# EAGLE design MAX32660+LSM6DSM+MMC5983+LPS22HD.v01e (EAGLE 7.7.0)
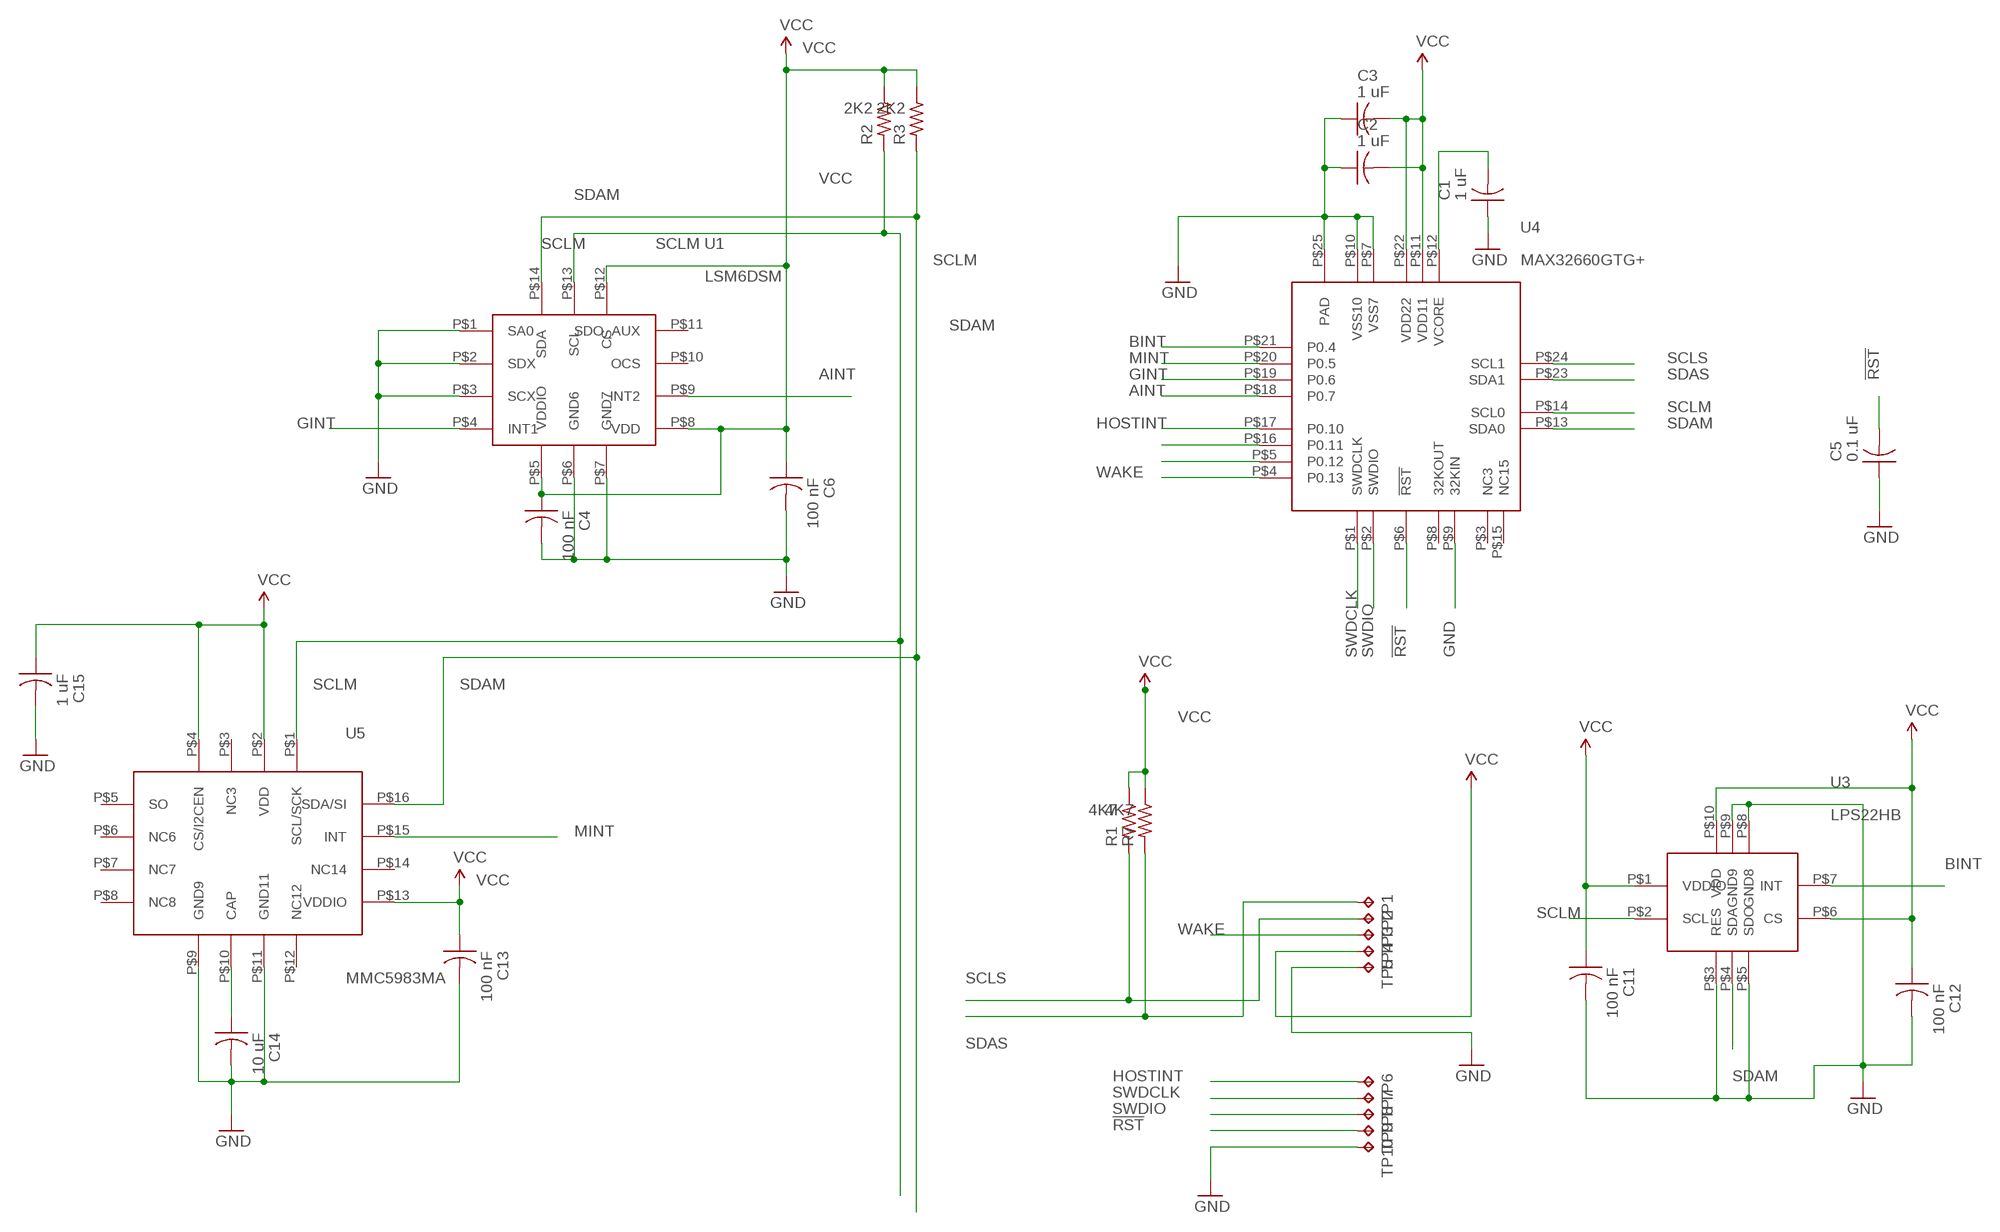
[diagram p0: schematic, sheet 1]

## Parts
C1  1 uF  C-US  [C0402_B]
C2  1 uF  C-US  [C0402_B]
C3  1 uF  C-US  [C0402_B]
C4  100 nF  C-US  [C0402_B]
C5  0.1 uF  C-US  [C0402_B]
C6  100 nF  C-US  [C0402_B]
C11  100 nF  C-US  [C0402_B]
C12  100 nF  C-US  [C0402_B]
C13  100 nF  C-US  [C0402_B]
C14  10 uF  C-US  [C0402_B]
C15  1 uF  C-US  [C0402_B]
R1  4K7  R-US_  [R0402_B]
R2  2K2  R-US_  [R0402_B]
R3  2K2  R-US_  [R0402_B]
R7  4K7  R-US_  [R0402_B]
TP1  TPTP08SQ  [TP08SQ]
TP2  TPTP08SQ  [TP08SQ]
TP3  TPTP08SQ  [TP08SQ]
TP4  TPTP08SQ  [TP08SQ]
TP5  TPTP08SQ  [TP08SQ]
TP6  TPTP08SQ  [TP08SQ]
TP7  TPTP08SQ  [TP08SQ]
TP8  TPTP08SQ  [TP08SQ]
TP9  TPTP08SQ  [TP08SQ]
TP10  TPTP08SQ  [TP08SQ]
U1  LSM6DSM  [LSM6DSM]
U3  LPS22HB  [LPS22HB]
U4  MAX32660GTG+  [MAX32660GTG+]
U5  MMC5983MA  [MMC5983MA]

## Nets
!RST: C5.2 TP9.TP U4.P$6(!RST)
AINT: U1.P$9(INT2) U4.P$18(P0.7)
BINT: U3.P$7(INT) U4.P$21(P0.4)
GINT: U1.P$4(INT1) U4.P$19(P0.6)
GND: C1.1 C2.1 C3.1 C4.2 C5.1 C6.2 C11.2 C12.2 C13.2 C14.2 C15.2 TP5.TP TP10.TP U1.P$1(SA0) U1.P$2(SDX) U1.P$3(SCX) U1.P$6(GND6) U1.P$7(GND7) U3.P$3(RES) U3.P$5(SDO) U3.P$8(GND8) U3.P$9(GND9) U4.P$7(VSS7) U4.P$9(32KIN) U4.P$10(VSS10) U4.P$25(PAD) U5.P$9(GND9) U5.P$11(GND11)
HOSTINT: TP6.TP U4.P$17(P0.10)
MINT: U4.P$20(P0.5) U5.P$15(INT)
N$2: C14.1 U5.P$10(CAP)
N$6: C1.2 U4.P$12(VCORE)
N$8: U4.P$16(P0.11)
N$9: U4.P$5(P0.12)
SCLM: R2.2 U1.P$13(SCL) U3.P$2(SCL) U4.P$14(SCL0) U5.P$1(SCL/SCK)
SCLS: R1.2 TP2.TP U4.P$24(SCL1)
SDAM: R3.2 U1.P$14(SDA) U3.P$4(SDA) U4.P$13(SDA0) U5.P$16(SDA/SI)
SDAS: R7.2 TP1.TP U4.P$23(SDA1)
SWDCLK: TP7.TP U4.P$1(SWDCLK)
SWDIO: TP8.TP U4.P$2(SWDIO)
VCC: C2.2 C3.2 C4.1 C6.1 C11.1 C12.1 C13.1 C15.1 R1.1 R2.1 R3.1 R7.1 TP4.TP U1.P$5(VDDIO) U1.P$8(VDD) U1.P$12(CS) U3.P$1(VDDIO) U3.P$6(CS) U3.P$10(VDD) U4.P$11(VDD11) U4.P$22(VDD22) U5.P$2(VDD) U5.P$4(CS/I2CEN) U5.P$13(VDDIO)
WAKE: TP3.TP U4.P$4(P0.13)
Unconnected: U4.P$3(NC3) U4.P$8(32KOUT) U4.P$15(NC15) U5.P$3(NC3) U5.P$5(SO) U5.P$6(NC6) U5.P$7(NC7) U5.P$8(NC8) U5.P$12(NC12) U5.P$14(NC14)

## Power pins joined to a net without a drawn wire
OCS: U1.P$10(OCS)
SDO_AUX: U1.P$11(SDO_AUX)

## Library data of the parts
C1-C6 C11-C15 = Spark:C-US: Capacitor
R1-R3 R7 = Spark:R-US_: 0402 Resistor
TP1-TP10 = testpad:TP: Test pad
U1 = Kris:LSM6DSM: LSM6DSM ST accel/gyro
U3 = Kris:LPS22HB: LPS22HB ST pressure sensor http://www.st.com/content/ccc/resource/technical/document/datasheet/bf/c1/4f/23/61/17/44/8a/DM00140895.pdf/files/DM00140895.pdf/jcr:content/translations/en.DM00140895.pdf
U4 = Kris:MAX32660GTG+: MAX32660GTG+ 3 mm x 3 mm 24-pin TQFN package https://pdfserv.maximintegrated.com/land_patterns/90-100089.PDF https://datasheets.maximintegrated.com/en/ds/MAX32660.pdf
U5 = Kris:MMC5983MA: MMC5983MA ±8 Gauss, High Performance 3-axis Magnetic Sensor https://www.mouser.com/datasheet/2/821/Memsic_09102019_MMC5983MA_Datasheet_Rev_A-1635338.pdf

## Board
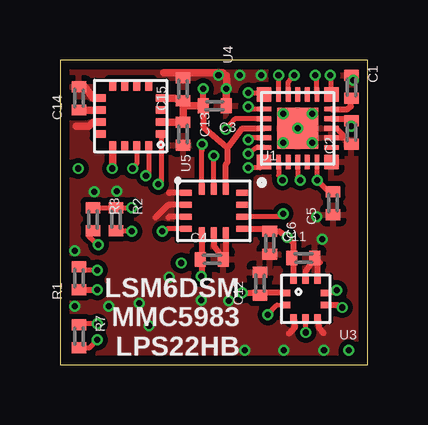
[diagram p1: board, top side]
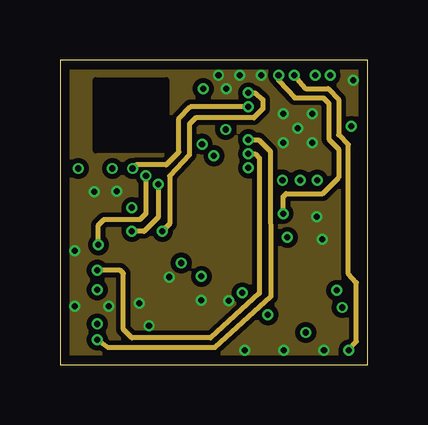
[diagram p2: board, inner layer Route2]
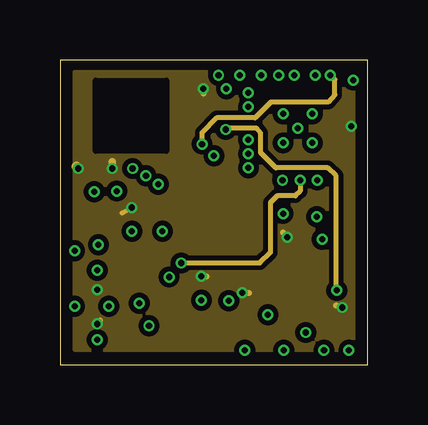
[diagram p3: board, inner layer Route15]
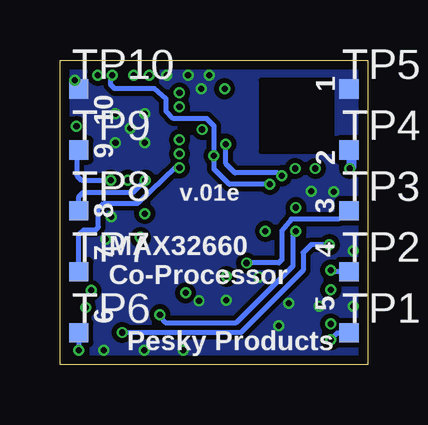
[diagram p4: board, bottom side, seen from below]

Size 12.83 x 12.7 mm. Coordinates in mm from the lower left corner, seen from the top.
Outline: 0,0 12.83,0 12.83,12.7 0,12.7 0,0
Copper layers (1*2*15*16): Top 0.035559375mm / dielectric 0.17018125mm / Route2 0.01778125mm / dielectric 47mil / Route15 0.01778125mm / dielectric 0.17018125mm / Bottom 0.035559375mm
Design rules "OSHPark-4layer *": minimum track width 5mil, minimum drill 10mil, track to track 5mil, track to pad 5mil, pad to pad 5mil, via to via 5mil, smd to smd 5mil, copper to edge 15mil, drill to drill 6mil, minimum pad ring 4mil, minimum via ring 4mil, stop-mask expansion 4mil, vias tented up to drill 20mil, thermal gap 10mil

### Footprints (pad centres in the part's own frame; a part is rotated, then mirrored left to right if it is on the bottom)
C0402_B = smd 0.457 x 0.61: 1 -0.483,0; 2 0.483,0
R0402_B = smd 0.457 x 0.61: 1 -0.483,0; 2 0.483,0
TP08SQ = smd 0.8 x 0.8: TP 0,0
LSM6DSM = smd 0.475 x 0.25: P$1 -1.163,0.75; P$2 -1.163,0.25; P$3 -1.163,-0.25; P$4 -1.163,-0.75; P$8 1.163,-0.75; P$9 1.163,-0.25; P$10 1.163,0.25; P$11 1.163,0.75 | smd 0.25 x 0.475: P$5 -0.5,-0.912; P$6 0,-0.912; P$7 0.5,-0.912; P$12 0.5,0.912; P$13 0,0.912; P$14 -0.5,0.912
LPS22HB = smd 0.3 x 0.275: P$1 -0.787,0.25; P$2 -0.787,-0.25; P$6 0.787,-0.25; P$7 0.787,0.25 | smd 0.275 x 0.3: P$3 -0.5,-0.787; P$4 0,-0.787; P$5 0.5,-0.787; P$8 0.5,0.787; P$9 0,0.787; P$10 -0.5,0.787
MAX32660GTG+ = smd 0.6 x 0.6: P$1 -1.4,1.4; P$7 -1.4,-1.4; P$13 1.4,-1.4; P$19 1.4,1.4 | smd 0.6 x 0.2: P$2 -1.4,0.8; P$3 -1.4,0.4; P$4 -1.4,0; P$5 -1.4,-0.4; P$6 -1.4,-0.8; P$14 1.4,-0.8; P$15 1.4,-0.4; P$16 1.4,0; P$17 1.4,0.4; P$18 1.4,0.8 | smd 0.2 x 0.6: P$8 -0.8,-1.4; P$9 -0.4,-1.4; P$10 0,-1.4; P$11 0.4,-1.4; P$12 0.8,-1.4; P$20 0.8,1.4; P$21 0.4,1.4; P$22 0,1.4; P$23 -0.4,1.4; P$24 -0.8,1.4 | smd 1.7 x 1.7: P$25 0,0
MMC5983MA = smd 0.3 x 0.45: P$1 0.75,1.275; P$2 0.25,1.275; P$3 -0.25,1.275; P$4 -0.75,1.275; P$9 -0.75,-1.275; P$10 -0.25,-1.275; P$11 0.25,-1.275; P$12 0.75,-1.275 | smd 0.45 x 0.3: P$5 -1.275,0.75; P$6 -1.275,0.25; P$7 -1.275,-0.25; P$8 -1.275,-0.75; P$13 1.275,-0.75; P$14 1.275,-0.25; P$15 1.275,0.25; P$16 1.275,0.75

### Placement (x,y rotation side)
C1  12.14,11.58 270 top
C2  12.14,9.68 90 top
C3  6.45,10.79 180 top
C4  6.32,4.39 0 top
C5  11.38,6.73 90 top
C6  8.74,5.08 270 top
C11  10.13,4.45 0 top
C12  8.33,3.38 90 top
C13  5.13,9.63 270 top
C14  0.79,11.1 90 top
C15  5.13,11.48 90 top
R1  0.79,3.61 90 top
R2  2.34,6.07 270 top
R3  1.37,6.07 270 top
R7  0.79,1.19 270 top
TP1  0.79,1.33 0 bottom
TP2  0.79,3.87 0 bottom
TP3  0.79,6.41 0 bottom
TP4  0.79,8.95 0 bottom
TP5  0.79,11.49 0 bottom
TP6  12.04,1.33 0 bottom
TP7  12.04,3.87 0 bottom
TP8  12.04,6.41 0 bottom
TP9  12.04,8.95 0 bottom
TP10  12.04,11.49 0 bottom
U1  6.41,6.41 0 top
U3  10.24,2.74 0 top
U4  9.91,9.86 90 top
U5  2.95,10.36 270 top

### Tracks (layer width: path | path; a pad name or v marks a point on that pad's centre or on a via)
!RST  (via drill 0.25)
  Top 0.203: U4.P$6 10.71,7.89 v10.72,7.7 11.2,7.21 C5.2
  Bottom 0.203: TP9.TP 12.13,8.97 12.13,7.89 11.94,7.7 v10.72,7.7
AINT  (via drill 0.25)
  Top 0.203: U4.P$18 v9.11,12.06 | v9.3,6.3 9.17,6.17 7.58,6.17 U1.P$9
  Route2 0.203: 9.4,6.3 v9.3,6.3 9.3,7.01 9.42,7.14 10.95,7.14 11.61,7.8 11.61,8.99 11.2,9.4 11.2,10.9 10.97,11.12 9.78,11.12 9.11,11.84 v9.11,12.06
BINT  (via drill 0.25)
  Top 0.203: U4.P$21 7.31,10.26 v6.91,9.8 | v11.53,3.1 11.53,3 11.18,3 11.18,2.99 U3.P$7
  Route15 0.203: v11.53,3.1 11.51,3.28 11.51,7.87 11.15,8.2 8.99,8.2 8.36,8.84 8.36,9.65 8.2,9.86 6.96,9.86 v6.91,9.8
GINT  (via drill 0.25)
  Top 0.203: U1.P$4 4.47,5.66 v4.27,5.56 | v7.85,11.33 8.38,11.33 U4.P$19
  Route2 0.203: v7.85,11.33 8.13,11.33 8.45,11.05 8.45,10.66 8.08,10.29 5.65,10.29 5.39,10.03 5.39,8.74 4.57,7.87 4.57,5.87 v4.27,5.56
GND  (via drill 0.25)
  Top 0.203: U4.P$9 11.91,9.46 | 10.85,4.27 C11.2 | U4.P$10 11.51,9.86 11.91,9.46 | 11.91,9.46 11.98,9.38 C2.1
  Top 0.254: U1.P$3 4.54,6.16 4.52,6.15 | 4.55,6.68 4.56,6.66 U1.P$2 4.5,6.66 3.99,6.15 | U1.P$1 4.57,7.16 4.55,7.19 | U1.P$6 6.41,4.97 C4.2 6.91,4.6 U1.P$7 | U3.P$9 10.24,3.89 C11.2 10.74,4.25 U3.P$8 | U3.P$5 10.79,1.56 10.97,1.32 | U3.P$3 9.79,1.56 9.55,1.29
  Top 0.305: U5.P$11 1.38,10.11 1.19,9.93 0.69,9.93 | C3.1 v6.93,11.51 6.96,11.53 6.93,12.04 6.78,12.17 5.18,12.17 5.13,11.94 | 0.76,11.53 C14.2 1.04,11.58 1.39,11.11 U5.P$9 | C15.2 5.13,11.99 5.1,12.17 4.32,12.17
  Top 0.406: C1.1 12.14,11.96 v12.22,11.86
  other vias: 9.3,9.25 10.52,9.25 9.3,10.46 10.52,10.46 9.91,9.86 11,0.61 3.3,2.57 3.71,1.63 7.04,2.67 5.89,2.69 7.7,0.61 9.32,0.61 0.61,2.44 0.61,4.75 4.55,3.66 2.03,2.44 10.92,5.23 10.69,6.17 2.36,7.24 1.42,7.21 8.38,12.06 7.49,12.06 6.6,12.06
  pour Bottom (isolate 0.203, no thermals): 0,12.7 12.83,12.7 12.83,0 0,0
  pour Route2 (isolate 0.203, no thermals): 0,12.7 12.83,12.7 12.83,0 0,0
  pour Top (isolate 0.203): 0,12.7 12.83,12.7 12.83,0 0,0
HOSTINT  (via drill 0.25)
  Top 0.203: U4.P$17 9.51,11.77 v9.75,12.06
  Route2 0.203: v9.75,12.06 10.24,11.51 11.18,11.51 11.61,11.05 11.61,9.58 12.01,9.17 12.01,3.79 12.34,3.43 12.34,0.96 12.04,0.64 v12.04,0.61
  Bottom 0.203: TP6.TP v12.04,0.61
MINT  (via drill 0.25)
  Top 0.203: U4.P$20 7.96,10.65 v7.85,10.74 | U5.P$15 3.2,8.38 v3.02,8.18
  Route2 0.203: v7.85,10.74 5.44,10.74 4.95,10.26 4.95,8.87 4.42,8.33 3.17,8.33 v3.02,8.18
N$2
  Top 0.305: U5.P$10 C14.1
N$3
  cutout Top: 9.3,3.73 11.28,3.73 11.28,1.78 9.3,1.78
N$4
  cutout Top: 1.47,11.86 4.45,11.86 4.45,8.89 1.47,8.89
  cutout Bottom: 1.47,11.86 4.45,11.86 4.45,8.89 1.47,8.89
  cutout Route15: 1.47,11.86 4.45,11.86 4.45,8.89 1.47,8.89
  cutout Route2: 1.47,11.89 4.45,11.89 4.45,8.92 1.47,8.92
N$5
  cutout Top: 4.88,7.7 7.95,7.7 7.95,5.16 4.88,5.16
N$6
  Top 0.254: U4.P$12 11.98,10.65 12.12,10.77 12.12,11.1 C1.2
SCLM  (via drill 0.25)
  Top 0.203: U1.P$13 v6.41,8.71 | v8.66,2.08 9.04,2.49 U3.P$2 | U4.P$14 10.71,11.98 v10.64,12.06 | v3,5.56 2.36,5.56 R2.2 | U5.P$1 4.22,7.65 v4.09,7.52
  Route2 0.203: v4.09,7.52 4.09,6.15 3.5,5.56 v3,5.56
  Bottom 0.203: v8.66,2.08 8.64,1.96 8.43,1.75 5.49,1.75 3.12,4.12 3.12,5.38 v3,5.56 | v10.64,12.06 10.71,11.98 10.71,11.66 10.55,11.51 8.89,11.51 8.41,11.07 8.41,10.57 8.1,10.26 6.71,10.26 6.41,9.96 v6.41,8.71 v6.4,8.7 6.4,8.15 5.77,7.52 v4.09,7.52
SCLS  (via drill 0.25)
  Top 0.203: U4.P$24 8.19,9.05 v7.85,8.79 | v1.55,3.94 1.04,3.94 R1.2
  Route2 0.203: v7.85,8.79 8.13,8.79 8.31,8.61 8.31,2.97 6.27,1.12 3,1.12 2.64,1.47 2.64,3.81 2.51,3.94 v1.55,3.94
  Bottom 0.203: TP2.TP 1.46,3.87 v1.55,3.94
SDAM  (via drill 0.25)
  Top 0.203: U1.P$14 5.91,8.92 v5.92,9.2 | v10.24,1.35 U3.P$4 | U4.P$13 11.3,12.01 v11.25,12.06 | R3.2 1.19,5.36 v1.6,5 | U5.P$16 3.7,7.96 v3.58,7.87
  Route2 0.203: v3.58,7.87 3.58,6.3 3.33,6.04 1.83,6.04 1.6,5.82 v1.6,5
  Route15 0.203: v11.25,12.06 11.46,11.88 11.46,11.25 11.18,10.95 8.79,10.95 8.13,10.29 6.53,10.29 5.92,9.68 v5.92,9.2
  Bottom 0.203: v10.24,1.35 5.28,1.35 2.69,3.94 2.69,4.67 2.36,5 v1.6,5 | v3.58,7.87 3.63,7.87 3.76,8 5.54,8 5.92,8.38 v5.92,9.2
SDAS  (via drill 0.25)
  Top 0.203: U4.P$23 7.91,9.46 v7.85,9.37 | R7.2 1.25,0.71 v1.55,1.04
  Route2 0.203: v7.85,9.37 8.28,9.37 8.76,8.89 8.79,2.85 6.45,0.71 2.01,0.71 v1.55,1.04
  Bottom 0.203: 0.83,1.33 1.29,1.32 | 1.29,1.32 v1.55,1.04 | 1.29,1.32 0.94,1.33 TP1.TP
SWDCLK  (via drill 0.25)
  Top 0.203: U4.P$1 8.33,8.2 v7.85,8.2
  Bottom 0.203: v7.85,8.2 8.03,8.2 9.52,6.78 9.59,6.73 11,6.73 11.23,6.5 11.23,5.74 11.34,5.62 11.82,5.62 12.04,5.41 TP7.TP
SWDIO  (via drill 0.25)
  Top 0.203: U4.P$2 9.11,7.89 v9.27,7.7
  Bottom 0.203: 9.25,7.62 v9.27,7.7 9.78,7.19 11.86,7.19 12.04,7.01 TP8.TP
VCC  (via drill 0.25)
  Top 0.203: v3,6.55 R2.1 R3.1 | v1.55,1.7 0.81,1.7 R7.1
  Top 0.254: U1.P$8 8.56,5.66 C6.1 9.14,5.56 v9.47,5.31 9.74,5.07 9.74,4.44 | 5.91,4.58 5.91,3.74 v5.89,3.68 | U1.P$5 5.91,4.58 | 5.91,4.58 C4.1 | U3.P$1 8.56,2.99 C12.1 8.23,3 v7.59,3 | 9.74,4.33 C11.1 9.74,4.44 | U3.P$6 11.55,2.49 v11.76,2.39 | R1.1 v1.55,3.12 | U4.P$11 11.94,10.26 C2.2 | U1.P$12 6.91,8.34 6.99,8.46 6.99,9.04 | 6.99,9.04 7.59,9.86 U4.P$22 | 6.99,9.04 6.93,9.09 5.97,9.91 C3.2 v5.97,11.51 | U3.P$10 9.74,4.33 | 9.74,4.33 9.74,4.44
  Top 0.305: 12.14,10.08 C2.2 | U5.P$13 2.2,8.29 2.16,8.23 v2.18,8.18 | U5.P$2 5,10.11 C13.1 C15.1 | U5.P$4 4.76,11.11 C15.1 | C3.2 5.18,10.79 C15.1
  Top 0.406: v12.14,9.93 12.14,10.08
  Route15 0.203: v3,6.55 2.59,6.33
  Route15 0.254: v5.89,3.68 6.1,3.68 | v7.59,3 7.87,3 | v9.47,5.31 9.3,5.51 | v11.76,2.39 11.68,2.39 11.51,2.46 | v1.55,1.7 1.68,1.85 | v1.55,3.12 1.65,3.17 | v5.97,11.51 5.97,11.3
  Route15 0.305: v2.18,8.18 2.18,8.46
  Route15 0.406: v0.76,8.18 0.69,8.26
  Bottom 0.406: TP4.TP 0.69,9.05 0.69,8.26 v0.76,8.18
  pour Route15 (isolate 0.203, no thermals): 0.63,12.19 12.19,12.19 12.19,0.64 0.63,0.64
WAKE  (via drill 0.25)
  Top 0.203: U4.P$4 9.91,7.8 v10.01,7.7
  Route15 0.203: v5.05,4.24 8.33,4.24 8.76,4.67 8.76,6.76 9.04,7.04 9.8,7.04 10.01,7.24 v10.01,7.7
  Bottom 0.203: 0.77,6.41 TP3.TP | TP3.TP 1.22,6.07 3.2,6.07 3.58,5.59 3.58,4.37 3.71,4.24 v5.05,4.24 | TP3.TP

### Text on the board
tPlace: LSM6DSM / MMC5983 / LPS22HB
bPlace: 1 | 10 | 2 | 9 | v.01e | 3 | 8 | 4 | 7 | 5 | MAX32660 / Co-Processor | 6 | Pesky Products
